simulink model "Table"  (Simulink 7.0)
settings: Solver=FixedStepDiscrete  SolverMode=SingleTasking  StartTime=0.0  StopTime=inf  FixedStep=samplePeriod  RelTol=1e-3  AbsTol=1e-6
PreLoadFcn:
  | initialize
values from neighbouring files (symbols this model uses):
  acal = acal(:)    [initialize.m]
  actParams = [	bulkModulus   * pressCanon    [initialize.m]
  dcal = dcal(:)    [initialize.m]
  fcal = fcal(:)    [initialize.m]
  forceCanon = 0.00444822    [initialize.m]    (also in TableInit.m = 1)
  inertia = inertia + inertiaP2Q([0 0 0], massA(i), cgA(:,i)-cg,  									inertiaCanon, massCanon)    [initialize.m]    (also in TableInit.m = [Ixx 0 0; 0 Iyy 0; 0 0 Izz])
  inertiaMask = zeros(3, 1)    [initialize.m]
  lengthCanon = 25.4    [initialize.m]    (also in TableInit.m)
  mass = ones(3, 1) * (sum(massA) + massT + massS)    [initialize.m]    (also in TableInit.m = 17300)
  massMask = zeros(3, 1)    [initialize.m]
  nTbl = length(dof)    [initialize.m]
  nUDPInp = nAct+nAcc+nAct    [initialize.m]
  nUDPOut = nAct    [initialize.m]
  returnPress = 50    [initialize.m]    (also in TableInit.m)
  rtg = cg    [initialize.m]    (also in TableInit.m = [0 0 cg])
  samplePeriod = controlPeriod/upsampleFactor    (= 0.00048828125)    [initialize.m]    (also in viewer.m = eval(getHeaderValue(header, 'DELTA_T')); TableInit.m = 0.0009765625)
  staticForce = forceT2A(ftbl, dtbl0, dof, rh, rb, rl, canon, atype)    [initialize.m]
  upsampleFactor = 2    [initialize.m]
undefined symbols (not defined in the file or in its folder): animation, atype, friction, yieldDispl
libraries: LibDynamics x12, LibTransforms x12

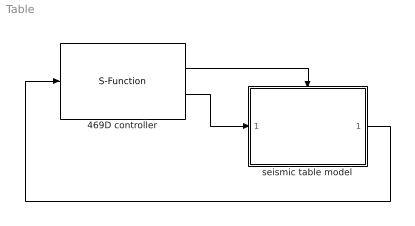
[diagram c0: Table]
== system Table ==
  469D controller : S-Function  FunctionName=UDPSimulink  Parameters=5002,nUDPInp,nUDPOut,upsampleFactor
  seismic table model : Subsystem  TreatAsAtomicUnit=on
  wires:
  469D controller/2 -> seismic table model/1(inp)
  469D controller/1 -> seismic table model/Trigger
  seismic table model/1(out) -> 469D controller/1

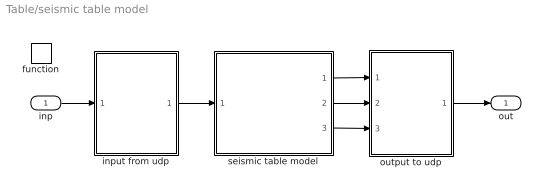
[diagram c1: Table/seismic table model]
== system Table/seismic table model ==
  inp : Inport  OutDataType=sfix(16)  OutScaling=2^0
  function : TriggerPort  TriggerType=function-call
  input from udp : Subsystem
  output to udp : Subsystem
  seismic table model : Subsystem
  out : Outport  OutDataType=sfix(16)  OutScaling=2^0
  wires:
  input from udp/1(valve cmd) -> seismic table model/1(valve cmd)
  inp/1 -> input from udp/1(inp)
  output to udp/1(out) -> out/1
  seismic table model/1(displ) -> output to udp/1(displ fbk)
  seismic table model/2(accel) -> output to udp/2(accel fbks)
  seismic table model/3(force) -> output to udp/3(force fbk)

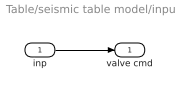
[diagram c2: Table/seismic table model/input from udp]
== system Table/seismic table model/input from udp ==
  inp : Inport  OutDataType=sfix(16)  OutScaling=2^0
  valve cmd : Outport  OutDataType=sfix(16)  OutScaling=2^0
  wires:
  inp/1 -> valve cmd/1

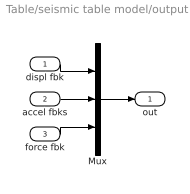
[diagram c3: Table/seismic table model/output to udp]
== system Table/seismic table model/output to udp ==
  displ fbk : Inport  OutDataType=sfix(16)  OutScaling=2^0
  accel fbks : Inport  Port=2  OutDataType=sfix(16)  OutScaling=2^0
  force fbk : Inport  Port=3  OutDataType=sfix(16)  OutScaling=2^0
  Mux : Mux  Inputs=3
  out : Outport  OutDataType=sfix(16)  OutScaling=2^0
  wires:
  force fbk/1 -> Mux/3
  accel fbks/1 -> Mux/2
  Mux/1 -> out/1
  displ fbk/1 -> Mux/1

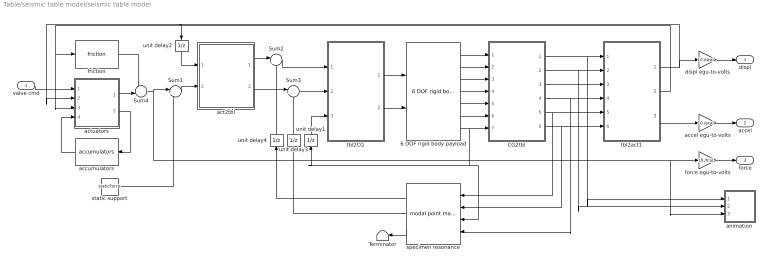
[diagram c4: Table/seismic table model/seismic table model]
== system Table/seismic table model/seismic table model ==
  valve cmd : Inport  OutDataType=sfix(16)  OutScaling=2^0
  6 DOF rigid body payload : LibDynamics/6 DOF rigid body payload  SystemSampleTime=-1  mass=mass.*massMask  inertia=diag(inertia.*inertiaMask)  gee=gee  massCanon=massCanon  inertiaCanon=inertiaCanon  linVelocCanon=linVelocCanon  linAccelCanon=linAccelCanon  rotDisplCanon=rotDisplCanon  rotVelocCanon=rotVelocCanon  rotAccelCanon=rotAccelCanon  rotForceCanon=rotForceCanon  initialPosition=zeros(6,1)  samplePeriod=samplePeriod
  CG2tbl : Subsystem  mask{ofst=-rtg}
      mask prompts: ofst "Origin offset"
  Sum1 : Sum  Inputs=|++  OutDataType=sfix(16)  OutScaling=2^0
  Sum2 : Sum  Inputs=|+-  OutDataType=sfix(16)  OutScaling=2^0
  Sum3 : Sum  Inputs=|+-  OutDataType=sfix(16)  OutScaling=2^0
  Sum4 : Sum  Inputs=-+|  OutDataType=sfix(16)  OutScaling=2^0
  Terminator : Terminator
  accel egu-to-volts : Gain  Gain=10./acal  ParameterDataType=sfix(16)  ParameterScaling=2^0  OutDataType=sfix(16)  OutScaling=2^0
  accumulators : LibDynamics/accumulators  Orientation=left  SystemSampleTime=-1  pumpFlow=pumpFlow  supplyPressure=supplyPress  precharge=precharge  bottleVolume=volume  gasConstant=gasConstant  flowCanon=flowCanon  volumeCanon=volumeCanon  samplePeriod=samplePeriod
  act2tbl : Subsystem
  actuators : Subsystem
  animation : Subsystem  mask{azim=-37.5, elev=35, params=animation, decim=ceil((1/samplePeriod)/32), samplePeriod=-1}
      mask prompts: azim "View azimuth (degrees)"; elev "View elevation (degrees)"; params "Parameters"; decim "Decimation factor"; samplePeriod "Sample period (sec)"
  displ egu-to-volts : Gain  Gain=10./dcal  ParameterDataType=sfix(16)  ParameterScaling=2^0  OutDataType=sfix(16)  OutScaling=2^0
  force egu-to-volts : Gain  Gain=10./fcal  ParameterDataType=sfix(16)  ParameterScaling=2^0  OutDataType=sfix(16)  OutScaling=2^0
  friction : LibDynamics/friction  SystemSampleTime=-1  friction=friction * forceCanon  yieldDispl=yieldDispl * lengthCanon  hysteresis=0  velocCanon=linVelocCanon  samplePeriod=samplePeriod
  specimen resonance : LibDynamics/modal point mass  Orientation=left  SystemSampleTime=-1  mass=modalMass  freq=modalFreq  damp=modalDamp  ofst=modalCG  gee=gee  massCanon=massCanon  linAccelCanon=linAccelCanon  rotDisplCanon=rotDisplCanon  rotVelocCanon=rotVelocCanon  rotForceCanon=rotForceCanon  samplePeriod=samplePeriod
  static support : Constant  Value=staticForce  OutDataType=sfix(16)  OutScaling=2^0
  tbl2CG : Subsystem  mask{ofst=rtg}
      mask prompts: ofst "Origin offset"
  tbl2act1 : Subsystem
  unit delay1 : UnitDelay  Orientation=up  X0=eye(3)  SampleTime=-1
  unit delay2 : UnitDelay  Orientation=down  SampleTime=-1
  unit delay3 : UnitDelay  Orientation=up  SampleTime=-1
  unit delay4 : UnitDelay  Orientation=up  SampleTime=-1
  displ : Outport  OutDataType=sfix(16)  OutScaling=2^0
  accel : Outport  Port=2  OutDataType=sfix(16)  OutScaling=2^0
  force : Outport  Port=3  OutDataType=sfix(16)  OutScaling=2^0
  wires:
  specimen resonance/3 -> Terminator/1
  static support/1 -> Sum1/2
  Sum1/1 -> act2tbl/2(force act)
  accel egu-to-volts/1 -> accel/1
  displ egu-to-volts/1 -> displ/1
  force egu-to-volts/1 -> force/1
  accumulators/1 -> actuators/4(press)
  actuators/2(flow) -> accumulators/1
  tbl2CG/2(force rpw) -> 6 DOF rigid body payload/2
  tbl2act1/1(displ act) -> unit delay2/1, actuators/2(displ), displ egu-to-volts/1
  valve cmd/1 -> actuators/1(cmds)
  tbl2CG/1(force xyz) -> 6 DOF rigid body payload/1
  6 DOF rigid body payload/1 -> CG2tbl/1(displ xyz)
  6 DOF rigid body payload/2 -> CG2tbl/2(displ rpw)
  6 DOF rigid body payload/3 -> CG2tbl/3(veloc xyz)
  6 DOF rigid body payload/4 -> CG2tbl/4(veloc rpw)
  6 DOF rigid body payload/5 -> CG2tbl/5(accel xyz)
  6 DOF rigid body payload/6 -> CG2tbl/6(accel rpw)
  6 DOF rigid body payload/7 -> CG2tbl/7(DCM), unit delay1/1, specimen resonance/3
  tbl2act1/3(accel act) -> accel egu-to-volts/1
  unit delay1/1 -> tbl2CG/3(DCM)
  unit delay2/1 -> act2tbl/1(displ act)
  tbl2act1/2(veloc act) -> actuators/3(veloc), friction/1
  CG2tbl/1(xyz) -> animation/1(xyz), tbl2act1/1(xyz)
  CG2tbl/2(rpw) -> animation/2(rpw), tbl2act1/2(rpw)
  CG2tbl/3(Vxyz) -> tbl2act1/3(Vxyz)
  CG2tbl/4(Vrpw) -> specimen resonance/4, tbl2act1/4(Vrpw)
  CG2tbl/5(Axyz) -> specimen resonance/1, tbl2act1/5(Axyz)
  CG2tbl/6(Arpw) -> specimen resonance/2, tbl2act1/6(Arpw)
  unit delay3/1 -> Sum3/2
  unit delay4/1 -> Sum2/2
  act2tbl/1(Fxyz) -> Sum2/1
  Sum2/1 -> tbl2CG/1(Fxyz)
  act2tbl/2(Frpw) -> Sum3/1
  Sum3/1 -> tbl2CG/2(Frpw)
  specimen resonance/1 -> unit delay4/1
  specimen resonance/2 -> unit delay3/1
  friction/1 -> Sum4/1
  actuators/1(force) -> Sum4/2
  Sum4/1 -> Sum1/1, force egu-to-volts/1, animation/3(Fact)

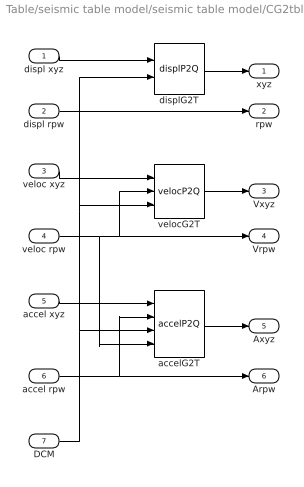
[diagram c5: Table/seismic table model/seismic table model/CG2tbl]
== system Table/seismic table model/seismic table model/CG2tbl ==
  displ xyz : Inport  OutDataType=sfix(16)  OutScaling=2^0
  displ rpw : Inport  Port=2  OutDataType=sfix(16)  OutScaling=2^0
  veloc xyz : Inport  Port=3  OutDataType=sfix(16)  OutScaling=2^0
  veloc rpw : Inport  Port=4  OutDataType=sfix(16)  OutScaling=2^0
  accel xyz : Inport  Port=5  OutDataType=sfix(16)  OutScaling=2^0
  accel rpw : Inport  Port=6  OutDataType=sfix(16)  OutScaling=2^0
  DCM : Inport  Port=7  OutDataType=sfix(16)  OutScaling=2^0
  accelG2T : LibTransforms/accelP2Q  SystemSampleTime=-1  dof=1:6  ofst=ofst
  displG2T : LibTransforms/displP2Q  SystemSampleTime=-1  dof=1:6  ofst=ofst
  velocG2T : LibTransforms/velocP2Q  SystemSampleTime=-1  dof=1:6  ofst=ofst
  xyz : Outport  OutDataType=sfix(16)  OutScaling=2^0
  rpw : Outport  Port=2  OutDataType=sfix(16)  OutScaling=2^0
  Vxyz : Outport  Port=3  OutDataType=sfix(16)  OutScaling=2^0
  Vrpw : Outport  Port=4  OutDataType=sfix(16)  OutScaling=2^0
  Axyz : Outport  Port=5  OutDataType=sfix(16)  OutScaling=2^0
  Arpw : Outport  Port=6  OutDataType=sfix(16)  OutScaling=2^0
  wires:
  accelG2T/1 -> Axyz/1
  velocG2T/1 -> Vxyz/1
  displ rpw/1 -> rpw/1
  displG2T/1 -> xyz/1
  displ xyz/1 -> displG2T/1
  accel xyz/1 -> accelG2T/1
  veloc xyz/1 -> velocG2T/1
  veloc rpw/1 -> Vrpw/1, velocG2T/2, accelG2T/4
  DCM/1 -> displG2T/2, velocG2T/3, accelG2T/3
  accel rpw/1 -> Arpw/1, accelG2T/2

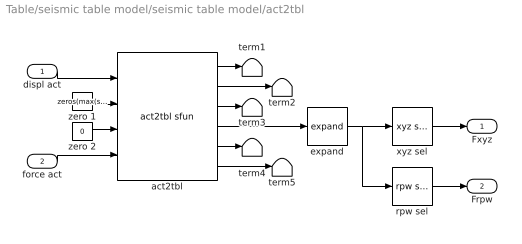
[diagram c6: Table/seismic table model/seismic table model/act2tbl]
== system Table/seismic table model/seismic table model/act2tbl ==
  displ act : Inport  OutDataType=sfix(16)  OutScaling=2^0
  force act : Inport  Port=2  OutDataType=sfix(16)  OutScaling=2^0
  act2tbl : LibTransforms/act2tbl sfun  atype=atype  nVel=0  nFrc=length(atype)  dof=dof  rh=rh  rb=rb  rl=rl  ra=[]  ea=[]  dmax=dmax  canon=canon  gee=gee  action=1  rate=0  count=1
  expand : LibTransforms/expand  SystemSampleTime=-1  size=6  elements=dof
  rpw sel : LibTransforms/rpw sel  SystemSampleTime=-1  dof=1:6
  term{1..5} (5 alike) : Terminator
  xyz sel : LibTransforms/xyz sel  SystemSampleTime=-1  dof=1:6
  zero 1 : Constant  Value=zeros(max(sum(dof>3), 1), 1)  OutDataType=sfix(16)  OutScaling=2^0
  zero 2 : Constant  Value=0  OutDataType=sfix(16)  OutScaling=2^0
  Fxyz : Outport  OutDataType=sfix(16)  OutScaling=2^0
  Frpw : Outport  Port=2  OutDataType=sfix(16)  OutScaling=2^0
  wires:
  expand/1 -> xyz sel/1, rpw sel/1
  act2tbl/6 -> term5/1
  act2tbl/5 -> term4/1
  act2tbl/3 -> term3/1
  act2tbl/2 -> term2/1
  act2tbl/1 -> term1/1
  zero 1/1 -> act2tbl/2
  zero 2/1 -> act2tbl/3
  act2tbl/4 -> expand/1
  displ act/1 -> act2tbl/1
  xyz sel/1 -> Fxyz/1
  force act/1 -> act2tbl/4
  rpw sel/1 -> Frpw/1

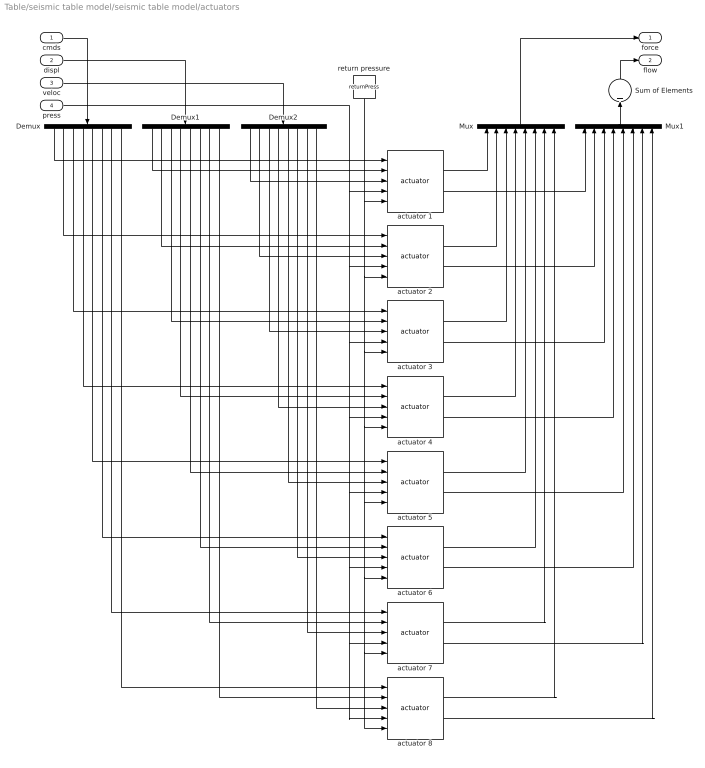
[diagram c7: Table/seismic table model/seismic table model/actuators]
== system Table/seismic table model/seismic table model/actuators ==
  cmds : Inport  OutDataType=sfix(16)  OutScaling=2^0
  displ : Inport  Port=2  OutDataType=sfix(16)  OutScaling=2^0
  veloc : Inport  Port=3  OutDataType=sfix(16)  OutScaling=2^0
  press : Inport  Port=4  OutDataType=sfix(16)  OutScaling=2^0
  Demux : Demux  Orientation=down  Outputs=nAct
  Demux1 : Demux  Orientation=down  Outputs=nAct
  Demux2 : Demux  Orientation=down  Outputs=nAct
  Mux : Mux  Orientation=up  Inputs=nAct
  Mux1 : Mux  Orientation=up  Inputs=nAct
  Sum of Elements : Sum  Orientation=up  Inputs=+  OutDataType=sfix(16)  OutScaling=2^-10
  actuator 1 : LibDynamics/actuator  SystemSampleTime=-1  params=actParams(:,1)
  actuator 2 : LibDynamics/actuator  SystemSampleTime=-1  params=actParams(:,2)
  actuator 3 : LibDynamics/actuator  SystemSampleTime=-1  params=actParams(:,3)
  actuator 4 : LibDynamics/actuator  SystemSampleTime=-1  params=actParams(:,4)
  actuator 5 : LibDynamics/actuator  SystemSampleTime=-1  params=actParams(:,5)
  actuator 6 : LibDynamics/actuator  SystemSampleTime=-1  params=actParams(:,6)
  actuator 7 : LibDynamics/actuator  SystemSampleTime=-1  params=actParams(:,7)
  actuator 8 : LibDynamics/actuator  SystemSampleTime=-1  params=actParams(:,8)
  return pressure : Constant  Orientation=down  Value=returnPress  OutDataType=sfix(16)  OutScaling=2^0
  force : Outport  OutDataType=sfix(16)  OutScaling=2^0
  flow : Outport  Port=2  OutDataType=sfix(16)  OutScaling=2^0
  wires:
  Sum of Elements/1 -> flow/1
  actuator 8/2 -> Mux1/8
  actuator 7/2 -> Mux1/7
  actuator 6/2 -> Mux1/6
  actuator 5/2 -> Mux1/5
  actuator 4/2 -> Mux1/4
  actuator 3/2 -> Mux1/3
  actuator 2/2 -> Mux1/2
  actuator 1/2 -> Mux1/1
  Mux1/1 -> Sum of Elements/1
  return pressure/1 -> actuator 1/5, actuator 2/5, actuator 3/5, actuator 4/5, actuator 5/5, actuator 6/5, actuator 8/5, actuator 7/5
  press/1 -> actuator 1/4, actuator 2/4, actuator 3/4, actuator 4/4, actuator 5/4, actuator 6/4, actuator 8/4, actuator 7/4
  veloc/1 -> Demux2/1
  actuator 8/1 -> Mux/8
  actuator 7/1 -> Mux/7
  actuator 6/1 -> Mux/6
  actuator 5/1 -> Mux/5
  actuator 4/1 -> Mux/4
  actuator 3/1 -> Mux/3
  actuator 2/1 -> Mux/2
  actuator 1/1 -> Mux/1
  Demux2/8 -> actuator 8/3
  Demux1/8 -> actuator 8/2
  Demux/8 -> actuator 8/1
  Demux2/7 -> actuator 7/3
  Demux1/7 -> actuator 7/2
  Demux/7 -> actuator 7/1
  Demux2/6 -> actuator 6/3
  Demux1/6 -> actuator 6/2
  Demux/6 -> actuator 6/1
  Demux2/5 -> actuator 5/3
  Demux1/5 -> actuator 5/2
  Demux/5 -> actuator 5/1
  Demux2/4 -> actuator 4/3
  Demux1/4 -> actuator 4/2
  Demux/4 -> actuator 4/1
  Demux2/3 -> actuator 3/3
  Demux1/3 -> actuator 3/2
  Demux/3 -> actuator 3/1
  Demux2/2 -> actuator 2/3
  Demux1/2 -> actuator 2/2
  Demux2/1 -> actuator 1/3
  Demux1/1 -> actuator 1/2
  Demux/2 -> actuator 2/1
  Demux/1 -> actuator 1/1
  displ/1 -> Demux1/1
  cmds/1 -> Demux/1
  Mux/1 -> force/1

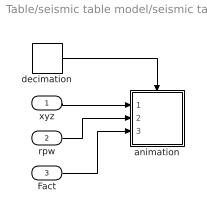
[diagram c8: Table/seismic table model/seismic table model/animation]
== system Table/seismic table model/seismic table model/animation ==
  xyz : Inport
  rpw : Inport  Port=2
  Fact : Inport  Port=3
  animation : Subsystem  TreatAsAtomicUnit=on
  decimation : DiscretePulseGenerator  Period=decim  SampleTime=samplePeriod
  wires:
  rpw/1 -> animation/2(rpw)
  Fact/1 -> animation/3(Fact)
  xyz/1 -> animation/1(xyz)
  decimation/1 -> animation/Trigger

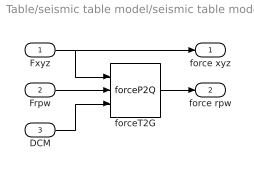
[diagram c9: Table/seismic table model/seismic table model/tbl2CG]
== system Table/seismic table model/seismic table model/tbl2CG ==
  Fxyz : Inport  OutDataType=sfix(16)  OutScaling=2^0
  Frpw : Inport  Port=2  OutDataType=sfix(16)  OutScaling=2^0
  DCM : Inport  Port=3  OutDataType=sfix(16)  OutScaling=2^0
  forceT2G : LibTransforms/forceP2Q  SystemSampleTime=-1  dof=1:6  ofst=ofst
  force xyz : Outport  OutDataType=sfix(16)  OutScaling=2^0
  force rpw : Outport  Port=2  OutDataType=sfix(16)  OutScaling=2^0
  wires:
  Frpw/1 -> forceT2G/2
  Fxyz/1 -> forceT2G/1, force xyz/1
  forceT2G/1 -> force rpw/1
  DCM/1 -> forceT2G/3

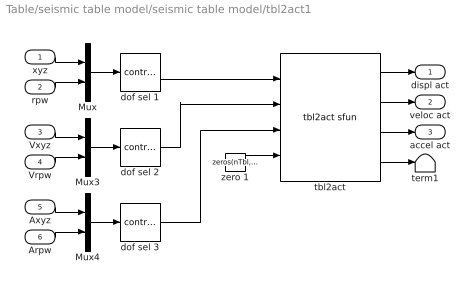
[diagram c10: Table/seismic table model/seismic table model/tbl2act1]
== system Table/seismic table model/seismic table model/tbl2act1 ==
  xyz : Inport  OutDataType=sfix(16)  OutScaling=2^0
  rpw : Inport  Port=2  OutDataType=sfix(16)  OutScaling=2^0
  Vxyz : Inport  Port=3  OutDataType=sfix(16)  OutScaling=2^0
  Vrpw : Inport  Port=4  OutDataType=sfix(16)  OutScaling=2^0
  Axyz : Inport  Port=5  OutDataType=sfix(16)  OutScaling=2^0
  Arpw : Inport  Port=6  OutDataType=sfix(16)  OutScaling=2^0
  Mux : Mux  Inputs=2
  Mux3 : Mux  Inputs=2
  Mux4 : Mux  Inputs=2
  dof sel 1 : LibTransforms/contract  SystemSampleTime=-1  elements=dof
  dof sel 2 : LibTransforms/contract  SystemSampleTime=-1  elements=dof
  dof sel 3 : LibTransforms/contract  SystemSampleTime=-1  elements=dof
  tbl2act : LibTransforms/tbl2act sfun  atype=atype  nVel=length(atype)  nFrc=0  dof=dof  rh=rh  rb=rb  rl=rl  ra=ra  ea=ea  offset=[0 0 0 0 0 0]  fmax=fmax  canon=canon  gee=gee  action=1  rate=0
  term1 : Terminator
  zero 1 : Constant  Value=zeros(nTbl, 1)  OutDataType=sfix(16)  OutScaling=2^0
  displ act : Outport  OutDataType=sfix(16)  OutScaling=2^0
  veloc act : Outport  Port=2  OutDataType=sfix(16)  OutScaling=2^0
  accel act : Outport  Port=3  OutDataType=sfix(16)  OutScaling=2^0
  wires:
  Mux4/1 -> dof sel 3/1
  Mux3/1 -> dof sel 2/1
  Mux/1 -> dof sel 1/1
  Arpw/1 -> Mux4/2
  Axyz/1 -> Mux4/1
  Vrpw/1 -> Mux3/2
  Vxyz/1 -> Mux3/1
  rpw/1 -> Mux/2
  xyz/1 -> Mux/1
  zero 1/1 -> tbl2act/4
  tbl2act/4 -> term1/1
  tbl2act/3 -> accel act/1
  tbl2act/2 -> veloc act/1
  tbl2act/1 -> displ act/1
  dof sel 1/1 -> tbl2act/1
  dof sel 2/1 -> tbl2act/2
  dof sel 3/1 -> tbl2act/3

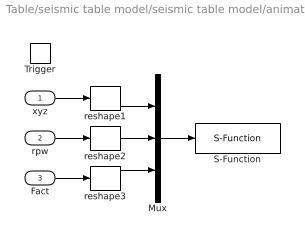
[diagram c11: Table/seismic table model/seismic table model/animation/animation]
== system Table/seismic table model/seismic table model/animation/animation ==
  xyz : Inport  OutDataType=sfix(16)  OutScaling=2^0
  rpw : Inport  Port=2  OutDataType=sfix(16)  OutScaling=2^0
  Fact : Inport  Port=3  OutDataType=sfix(16)  OutScaling=2^0
  Trigger : TriggerPort
  Mux : Mux  Inputs=3
  S-Function : S-Function  FunctionName=animation  Parameters=azim,elev,params
  reshape1 : Reshape
  reshape2 : Reshape
  reshape3 : Reshape
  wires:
  reshape1/1 -> Mux/1
  reshape2/1 -> Mux/2
  rpw/1 -> reshape2/1
  reshape3/1 -> Mux/3
  Fact/1 -> reshape3/1
  xyz/1 -> reshape1/1
  Mux/1 -> S-Function/1
